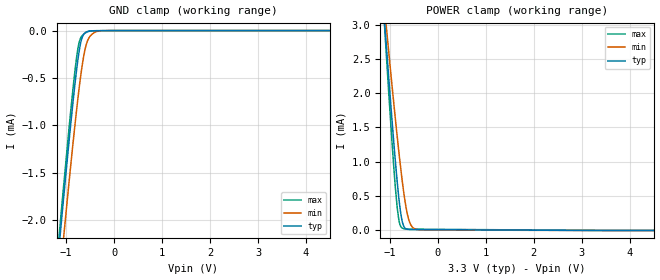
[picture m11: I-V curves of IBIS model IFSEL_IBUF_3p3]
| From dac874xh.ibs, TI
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|   IFSEL_IBUF_3p3 Model
[Model]   IFSEL_IBUF_3p3
Model_type   Input
Vinl = 0.99
Vinh =  2.31
|   typ   min   max
C_comp   1.45221E-13  3.61073E-14  2.15954E-13
| Where nom  PVT is Nominal Process, 3.3V, 27C
|   Fast PVT is Strong Process,  3.6V, -40C
|   Slow PVT is Weak Process,   3.0V, 150C
[Model spec]
|subparameter
Vinl   0.99   0.9   1.08
Vinh   2.31   2.1   2.52
[Voltage Range]   3.3   3   3.6
[Temperature Range]   27   150   -40
[Power Clamp Reference]   3.3   3   3.6
[GND Clamp Reference]   0   0   0
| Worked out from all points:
|   GND clamp passes 1 mA (typ) near -0.91 V on its own axis
|   POWER clamp passes 1 mA (typ) near -0.88 V on its own axis
[GND Clamp]
|   Voltage   I(typ)   I(min)   I(max)
-3.3V     -14.67mA   -14.74mA   -14.83mA
-1.251V   -2.855mA   -3.239mA   -2.753mA
-1.102V   -2.035mA   -2.444mA   -1.917mA
-1.053V   -1.767mA   -2.183mA   -1.643mA
-904.2mV  -987.9uA   -1.422mA   -849.3uA
-775.5mV  -389.1uA   -809.3uA   -260uA
-726mV    -210uA     -596.7uA   -120.6uA
-676.5mV  -90.17uA   -407.1uA   -60.71uA
-567.6mV  -12.25uA   -127.4uA   -16.12uA
-458.7mV  -2.332uA   -37.09uA   -3.113uA
-260.7mV  -857.4nA   -1.433uA   -1.163uA
6.6V      0A         0A         0A
[POWER Clamp]
|   Voltage   I(typ)   I(min)   I(max)
-3.3V     25.23mA    20.42mA    29.41mA
-1.112V   3.055mA    3.249mA    2.992mA
-1.092V   2.867mA    3.102mA    2.769mA
-1.023V   2.218mA    2.595mA    2.001mA
-933.9mV  1.416mA    1.96mA     1.072mA
-874.5mV  920.3uA    1.551mA    535.1uA
-805.2mV  423.8uA    1.098mA    127.7uA
-735.9mV  113uA      687.3uA    33.13uA
-666.6mV  24.92uA    351.9uA    21.61uA
-597.3mV  14.09uA    137.4uA    19.25uA
-399.3mV  12.32uA    10.67uA    18uA
6.6V      0A         0A         0A
